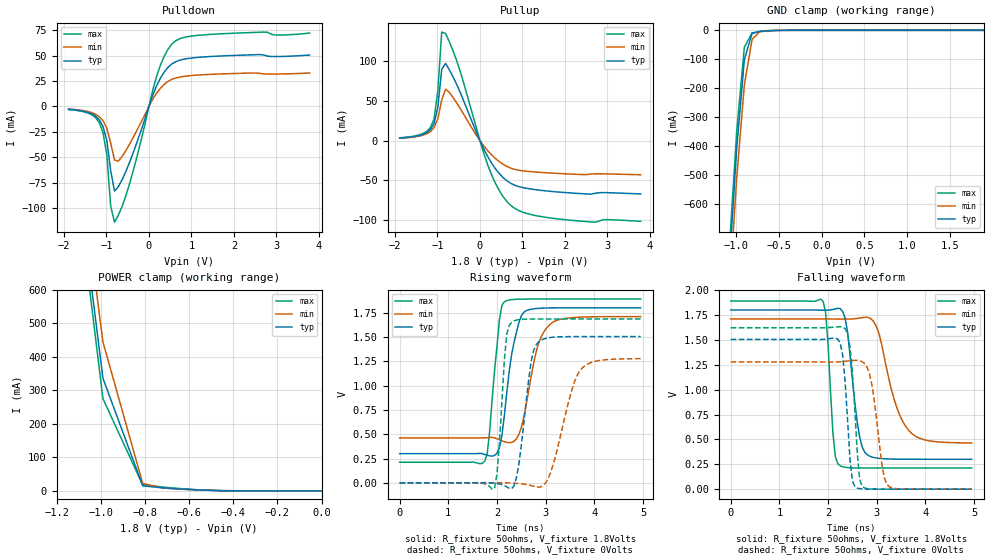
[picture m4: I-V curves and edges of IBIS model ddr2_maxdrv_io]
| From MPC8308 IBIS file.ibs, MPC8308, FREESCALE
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[Model]   ddr2_maxdrv_io   |
Model_type   I/O
Vinl = 0.87
Vinh = 0.93
Vmeas = 0.9
Cref = 1E-11
Rref = 50
Vref = 0.9
| variable   typ   min   max
C_comp   1.17p   1.10p   1.23p
[Model Spec]
| subparameter   typ   min   max
S_overshoot_high  3.300   3.135   3.465
S_overshoot_low   -200.00m  -100.00m  -300.00m
D_overshoot_high  4.000   4.000   4.000
D_overshoot_low   -1.000   -1.000   -1.000
D_overshoot_time  1.000n   1.000n   1.000n
| variable   typ   min   max
[Temperature Range]   25.0   -40.0   125.0
| variable   typ   min   max
[Pullup Reference]   1.800V   1.710V   1.890V
| variable   typ   min   max
[Pulldown Reference]   0.000V   0.000V   0.000V
| variable   typ   min   max
[POWER_Clamp_Reference]   1.800V   1.710V   1.890V
| variable   typ   min   max
[GND_Clamp_Reference]   0.000V   0.000V   0.000V
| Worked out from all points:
|   slope of the pulldown table from 0 to 0.27 V, typ, clamps not added: 9.72 ohm
|   slope of the pullup table from 0 to 0.27 V, typ, clamps not added: 9.65 ohm
|   GND clamp passes 1 mA (typ) near -0.59 V on its own axis
|   POWER clamp passes 1 mA (typ) near -0.47 V on its own axis
|   rising waveform, R_fixture 50ohms, V_fixture 1.8Volts: 20-80 % time 248ps typ, 309ps min, 175ps max; typ from 0.3 V to 1.8 V
|   rising waveform, R_fixture 50ohms, V_fixture 0Volts: 20-80 % time 212ps typ, 389ps min, 129ps max; typ from 0 V to 1.5 V
|   falling waveform, R_fixture 50ohms, V_fixture 1.8Volts: 20-80 % time 206ps typ, 402ps min, 119ps max; typ from 1.8 V to 0.3 V
|   falling waveform, R_fixture 50ohms, V_fixture 0Volts: 20-80 % time 123ps typ, 195ps min, 130ps max; typ from 1.5 V to 0 V
[Pulldown]
| pulldown in the table = pulldown subtract gnd_clamp
|Voltage   I(typ)   I(min)   I(max)
-1.89V    -2.91mA    -2.604mA   -3.068mA
-1.17V    -13.04mA   -10.01mA   -15.74mA
-1.08V    -19.79mA   -14.08mA   -25.82mA
-990mV    -33.63mA   -21.56mA   -48.01mA
-900mV    -63.16mA   -35.96mA   -97.93mA
-810mV    -83.34mA   -52.8mA    -114mA
-720mV    -79.09mA   -53.84mA   -107.1mA
-450mV    -54.49mA   -36.83mA   -75.29mA
180mV     20.2mA     12.97mA    29.38mA
540mV     41.79mA    26.63mA    61.34mA
1.26V     48.6mA     31.13mA    70.31mA
3.78V     50.58mA    32.89mA    72.17mA
[Pullup]
| pullup in the table = pullup subtract power_clamp
|Voltage   I(typ)   I(min)   I(max)
-1.89V    3.327mA    3.037mA    3.614mA
-1.35V    7.777mA    6.757mA    8.801mA
-1.08V    21.52mA    16.42mA    27.18mA
-990mV    42.64mA    27.73mA    63.15mA
-900mV    89.69mA    51.18mA    136.8mA
-810mV    97.42mA    64.89mA    135.2mA
-720mV    89.28mA    60.85mA    124.5mA
-450mV    59.07mA    39.32mA    84.77mA
270mV     -27.97mA   -17.75mA   -42.6mA
720mV     -53.64mA   -34.51mA   -81.38mA
1.71V     -64.11mA   -40.95mA   -97.79mA
3.78V     -67.14mA   -43mA      -101.6mA
[GND_clamp]
|Voltage   I(typ)   I(min)   I(max)
-1.89V    -5.289A    -5.314A    -5.291A
-1.08V    -830.5mA   -924.5mA   -780.6mA
-990mV    -411.5mA   -514.7mA   -352.7mA
-900mV    -101.5mA   -188.4mA   -58.29mA
-810mV    -10.46mA   -31.1mA    -8.864mA
-720mV    -3.532mA   -4.591mA   -4.66mA
-630mV    -1.451mA   -1.339mA   -1.97mA
1.89V     11.74nA    4.438uA    11.9pA
[POWER_clamp]
|Voltage   I(typ)   I(min)   I(max)
-1.71V    4.942A     4.957A     4.954A
-1.08V    811.3mA    908.1mA    762.8mA
-990mV    336.3mA    444.6mA    275.5mA
-810mV    15.09mA    22.51mA    17.99mA
-720mV    9.216mA    8.568mA    11.65mA
-630mV    5.341mA    4.938mA    6.448mA
-450mV    673.8uA    1mA        542.4uA
0V        210.7pA    7.657nA    11.9pA
[Ramp]
|Voltage   I(typ)   I(min)   I(max)
dV/dt_f   0.91/204.464p 0.76/405.823p 1.02/116.045p
dV/dt_r   0.94/219.664p 0.79/403.799p 1.05/129.742p
R_load=50ohms
| R_load was connected to ground for Ramp_up test and power for Ramp_dn test
[Rising_Waveform]
R_fixture=50ohms
V_fixture=1.8Volts
V_fixture_min=1.71Volts
V_fixture_max=1.89Volts
|C_fixture=1E-15f
|L_fixture=1E-15h
|C_dut=1E-15fh
|R_dut=0.001ohm
|L_dut=1E-12h
|time   V(typ)   V(min)   V(max)
0s        300.4mV    463.1mV    211.8mV
1.75ns    291.9mV    463.2mV    224.2mV
1.85ns    277.3mV    467.1mV    534.7mV
2ns       305.8mV    453.6mV    1.408V
2.15ns    687.9mV    423.7mV    1.862V
2.3ns     1.32V      416.3mV    1.884V
2.55ns    1.754V     673.8mV    1.89V
2.85ns    1.794V     1.43V      1.89V
3.1ns     1.799V     1.635V     1.89V
4.95ns    1.8V       1.71V      1.89V
[Rising_Waveform]
R_fixture=50ohms
V_fixture=0Volts
|C_fixture=1E-15f
|L_fixture=1E-15h
|C_dut=1E-15fh
|R_dut=0.001ohm
|L_dut=1E-12h
|time   V(typ)   V(min)   V(max)
0s        4.791nV    470.6nV    54.98pV
1.95ns    -3.55mV    1.842mV    -55.48mV
2.2ns     -40.56mV   1.011mV    1.529V
2.3ns     -60.13mV   -1.301mV   1.65V
2.45ns    198.4mV    -7.247mV   1.679V
2.7ns     1.245V     -27.69mV   1.685V
2.85ns    1.447V     -44.23mV   1.686V
3.1ns     1.495V     106mV      1.686V
3.7ns     1.504V     1.151V     1.686V
4.95ns    1.505V     1.277V     1.686V
[Falling_Waveform]
R_fixture=50ohms
V_fixture=1.8Volts
V_fixture_min=1.71Volts
V_fixture_max=1.89Volts
|C_fixture=1E-15f
|L_fixture=1E-15h
|C_dut=1E-15fh
|R_dut=0.001ohm
|L_dut=1E-12h
|time   V(typ)   V(min)   V(max)
0s        1.8V       1.71V      1.89V
1.9ns     1.798V     1.71V      1.885V
1.95ns    1.798V     1.71V      1.776V
2.15ns    1.811V     1.709V     325.3mV
2.25ns    1.814V     1.708V     234.5mV
2.4ns     1.584V     1.708V     216.8mV
2.75ns    373.8mV    1.726V     212.1mV
3ns       312.5mV    1.627V     211.9mV
3.65ns    300.7mV    594.2mV    211.8mV
4.95ns    300.4mV    464.2mV    211.8mV
[Falling_Waveform]
R_fixture=50ohms
V_fixture=0Volts
|C_fixture=1E-15f
|L_fixture=1E-15h
|C_dut=1E-15fh
|R_dut=0.001ohm
|L_dut=1E-12h
|time   V(typ)   V(min)   V(max)
0s        1.505V     1.278V     1.621V
2.15ns    1.517V     1.277V     1.629V
2.3ns     1.347V     1.282V     1.63V
2.5ns     84.9mV     1.292V     1.179V
2.6ns     10.41mV    1.294V     361mV
2.7ns     3.121mV    1.28V      29.14mV
2.9ns     703.9uV    1.05V      1.593mV
3.1ns     204.6uV    266.6mV    343.2uV
3.25ns    84.52uV    27.21mV    112.1uV
4.95ns    -11.51nV   11.38uV    -3.36nV
